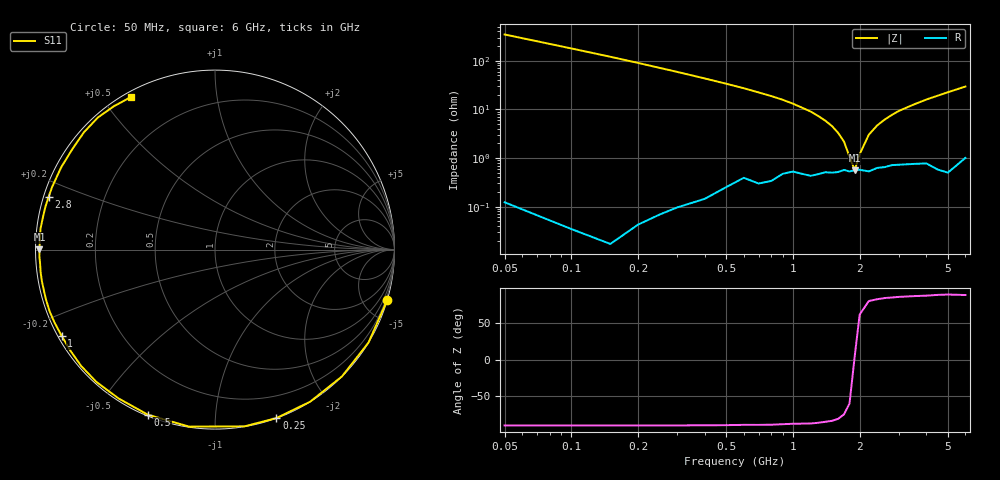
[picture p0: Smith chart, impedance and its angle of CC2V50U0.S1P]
! Infineon Technologies  Discrete & RF Semiconductors
! BBY57-02W
! Si Tuning Diode in SCD-80
! VR = 2.5 V
! S-Parameters:  June  2000
# GHz  S  MA  R  50
!  f  S11
! GHz  MAG  ANG
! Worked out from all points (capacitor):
!   34 points, 50 MHz to 6 GHz, reference 50 ohm
!   read as one part to ground: C = 8.86 pF near 50 MHz
!   lowest |Z| = 563 mohm at 1.9 GHz (marker M1)
!   series resonance near 1.895 GHz, so ESL is about 800 pH
!   S11 on the Smith chart (normalised r, x): 50 MHz: 0.00, -6.94; 250 MHz: 0.00, -1.43; 500 MHz: 0.01, -0.67; 1 GHz: 0.01, -0.26; 2.8 GHz: 0.01, +0.15; 6 GHz: 0.02, +0.59
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0.05  0.9999 -16.4
0.1  0.9999 -31.2
0.15  0.9999 -45.0
0.2  0.9996 -58.0
0.25  0.9991 -70.0
0.3  0.9984 -80.5
0.4  0.9967 -98.3
0.5  0.9931 -112.1
0.6  0.988 -122.9
0.7  0.9901 -131.9
0.8  0.9882 -139.0
0.9  0.9829 -145.1
1  0.9805 -150.7
1.1  0.9821 -155.6
1.3  0.982 -163.4
1.6  0.9797 -172.6
1.8  0.9791 -177.9
1.9  0.9778 179.9
2.2  0.9791 173.2
2.4  0.9755 169.4
2.8  0.9725 162.5
3  0.9723 159.1
3.5  0.972 151.9
4  0.9723 144.7
4.5  0.98 138.2
5  0.9835 131.6
5.5  0.9776 125.3
6  0.9706 119.0
